FUNCTION_BLOCK FB75
TITLE =Set Position Profile
//*****************************************************************************
//* maxon motor ag
//* R&D
//* all rights reserved
//*****************************************************************************
//* Summary:  Set position profile
//*
//* Remarks:
//*
//* Created under: STEP7 REV5.2+SP1
//*****************************************************************************
//* History:
//* 18.05.2004 | INA   first release
//*
//*
//*****************************************************************************
//

AUTHOR:INA
FAMILY:ProPosMo
NAME:SetPosPr
VERSION:00.01


VAR_INPUT

Write : BOOL //A rising edge start the command

  NodeID : BYTE //Adress of the maxon device

  ProfileVelocity : DWORD //Position Profile Velocity

  ProfileAcceleration : DWORD //Position Profile Acceleration

  ProfileDeceleration : DWORD //Position Profile Deceleration

END_VAR
VAR_OUTPUT
  Done : BOOL //Data valid flag is TRUE if data were available

  Err : BOOL //Error flag is TRUE if an Error has occured, see ErrNo for more details

  ErrNo : DINT //Contains detailed error information

END_VAR
VAR
  xEdgeMerker : BOOL //Edge Merker

  xEdgeFlag : BOOL //Edge Flag

  xStep : INT
END_VAR

BEGIN

NETWORK
TITLE = Activate the service function
//

// SDO Write "Set Position Profile"

       U    #Write
       FP   #xEdgeFlag                   // recognize a positiv edge of the Read signal
       =    #xEdgeMerker                 // and set the xEdgeMerker for one cycle to true

       L    #xStep
       L    0
       ==I
       U    #xEdgeMerker
       SPB  nstp                         // iStep = 1 -> fnc1

       L    #xStep                       // jump list
       SPL  List
       SPA  rdef
       SPA  fnc1
       SPA  fncE
List  :SPA  rdef

rdef  :NOP  0
       R    #Done                        // reset Done
       R    #Err
       L    0
       T    #xStep                       // iStep = 0
       SPA  end

fnc1  :NOP  0
       CALL FC16
         NodeID:=#NodeID
         Index:=DW#16#00006081
         SubIndex:=DW#16#00000000
         ValueIn:=#ProfileVelocity
         RET_VAL:=#Done
         Err:=#Err
         ErrNo:=#ErrNo

       L    1
       U    #Err
       SPB  fncE

       NOP  0
       CALL FC16
         NodeID:=#NodeID
         Index:=DW#16#00006083
         SubIndex:=DW#16#00000000
         ValueIn:=#ProfileAcceleration
         RET_VAL:=#Done
         Err:=#Err
         ErrNo:=#ErrNo

       L    1
       U    #Err
       SPB  fncE

       NOP  0
       CALL FC16
         NodeID:=#NodeID
         Index:=DW#16#00006084
         SubIndex:=DW#16#00000000
         ValueIn:=#ProfileDeceleration
         RET_VAL:=#Done
         Err:=#Err
         ErrNo:=#ErrNo

       L    1
       U    #Err
       SPB  fncE

       SPA  nstp                         // iStep = 3 -> fncE

fncE  :NOP  0
       L    0
       T    #xStep
       SPA  end

nstp  :NOP  0
       L    #xStep
       INC            1
       T    #xStep

end   :NOP  0
END_FUNCTION_BLOCK
